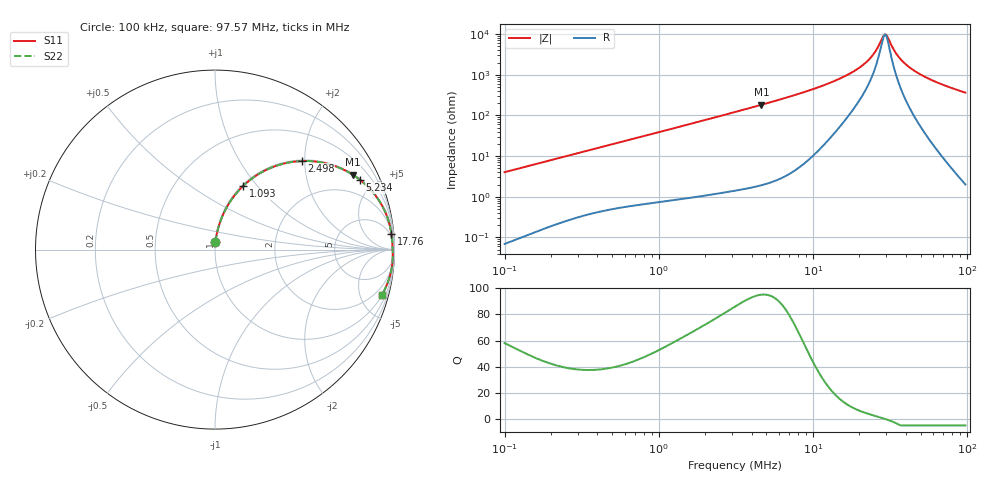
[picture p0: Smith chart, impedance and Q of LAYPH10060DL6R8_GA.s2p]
! LAYPH10060DL6R8_GA  S-PARAMETER MODEL  ( General Type )
! Model Generated by TAIYO YUDEN Corporation (http://www.ty-top.com)
! Version 3.0
! TAIYO YUDEN Control No. 180828NI43SB-FBB
! Copyright(c) 2017 TAIYO YUDEN CO.,LTD. All Rights Reserved.
! Product Description (link to TY-COMPAS)
! https://ds.yuden.co.jp/TYCOMPAS/or/detail?pn=LAYPH10060DL6R8NGA&u=M
! Products Name : Inductors
! Characteristics :
!  Inductance : 6.8 uH , SRF(min) : -Hz , DC Resistance(max) : 0.021 Ohm
!  Rated Current : Saturation :5.5 A , Temp Rise : 3.5 A (25 degC)
!  Case Size : 10.1 x 10.0 / 0.398 x 0.394 [mm/inch] , Thickness : 6 / 0.236 [mm/inch]
!  (Conditions: Temperature = 25 degC , DC Bias Current/Voltage = 0A / 0V)
! External Node Assignments :
!  1  o---GGG---o  2
! GND o---------o GND
! Frequency Range : 0.1MHz  -  97.572838MHz  [ 402 STEP ]
# MHz S RI R 50
! Freq[MHz].  S11 Real  S11 Imag  S21 Real  S21 Imag  S12 Real  S12 Imag  S22 Real  S22 Imag
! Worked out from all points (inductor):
!   401 points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, 100 kHz to 97.57 MHz, reference 50 ohm
!   read as one part in series: L = 6.38 uH near 103.5 kHz
!   highest Q = 95.1 at 4.64 MHz (marker M1), where L = 6.26 uH
!   self-resonance near 29.25 MHz
!   S11 on the Smith chart (normalised r, x): 100 kHz: 1.00, +0.08; 1.093 MHz: 1.02, +0.84; 2.498 MHz: 1.02, +1.93; 5.234 MHz: 1.04, +4.15; 17.76 MHz: 3, +22; 97.57 MHz: 1.04, -7.26
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0.1  0.0023 0.0401  0.9977 -0.0401  0.9977 -0.0401  0.0023 0.0401
0.316747  0.0185 0.1222  0.9815 -0.1222  0.9815 -0.1222  0.0185 0.1222
1.003287  0.1353 0.3327  0.8647 -0.3327  0.8647 -0.3327  0.1353 0.3327
1.093432  0.1558 0.3537  0.8442 -0.3537  0.8442 -0.3537  0.1558 0.3537
1.596632  0.2779 0.4404  0.7221 -0.4404  0.7221 -0.4404  0.2779 0.4404
2.497533  0.4823 0.4934  0.5177 -0.4934  0.5177 -0.4934  0.4823 0.4934
3.177882  0.6019 0.4838  0.3981 -0.4838  0.3981 -0.4838  0.6019 0.4838
4.640352  0.767 0.4175  0.233 -0.4175  0.233 -0.4175  0.767 0.4175
5.234367  0.8092 0.3877  0.1908 -0.3877  0.1908 -0.3877  0.8092 0.3877
9.894118  0.9456 0.2159  0.0544 -0.2159  0.0544 -0.2159  0.9456 0.2159
17.76111  0.9829 0.0863  0.0171 -0.0863  0.0171 -0.0863  0.9829 0.0863
20.73624  0.986 0.0583  0.014 -0.0583  0.014 -0.0583  0.986 0.0583
23.3907  0.9877 0.0378  0.0123 -0.0378  0.0123 -0.0378  0.9877 0.0378
25.49235  0.9887 0.0236  0.0113 -0.0236  0.0113 -0.0236  0.9887 0.0236
28.75564  0.9898 0.00364  0.0102 -0.00364  0.0102 -0.00364  0.9898 0.00364
29.76252  0.99 -0.00209  0.00997 0.00209  0.00997 0.00209  0.99 -0.00209
31.33933  0.9903 -0.0108  0.00968 0.0108  0.00968 0.0108  0.9903 -0.0108
33.57244  0.9905 -0.0225  0.00946 0.0225  0.00946 0.0225  0.9905 -0.0225
36.58892  0.9905 -0.0376  0.00953 0.0376  0.00953 0.0376  0.9905 -0.0376
44.98103  0.9881 -0.0759  0.0119 0.0759  0.0119 0.0759  0.9881 -0.0759
62.37672  0.9752 -0.1443  0.0248 0.1443  0.0248 0.1443  0.9752 -0.1443
97.57284  0.9283 -0.2553  0.0717 0.2553  0.0717 0.2553  0.9283 -0.2553
